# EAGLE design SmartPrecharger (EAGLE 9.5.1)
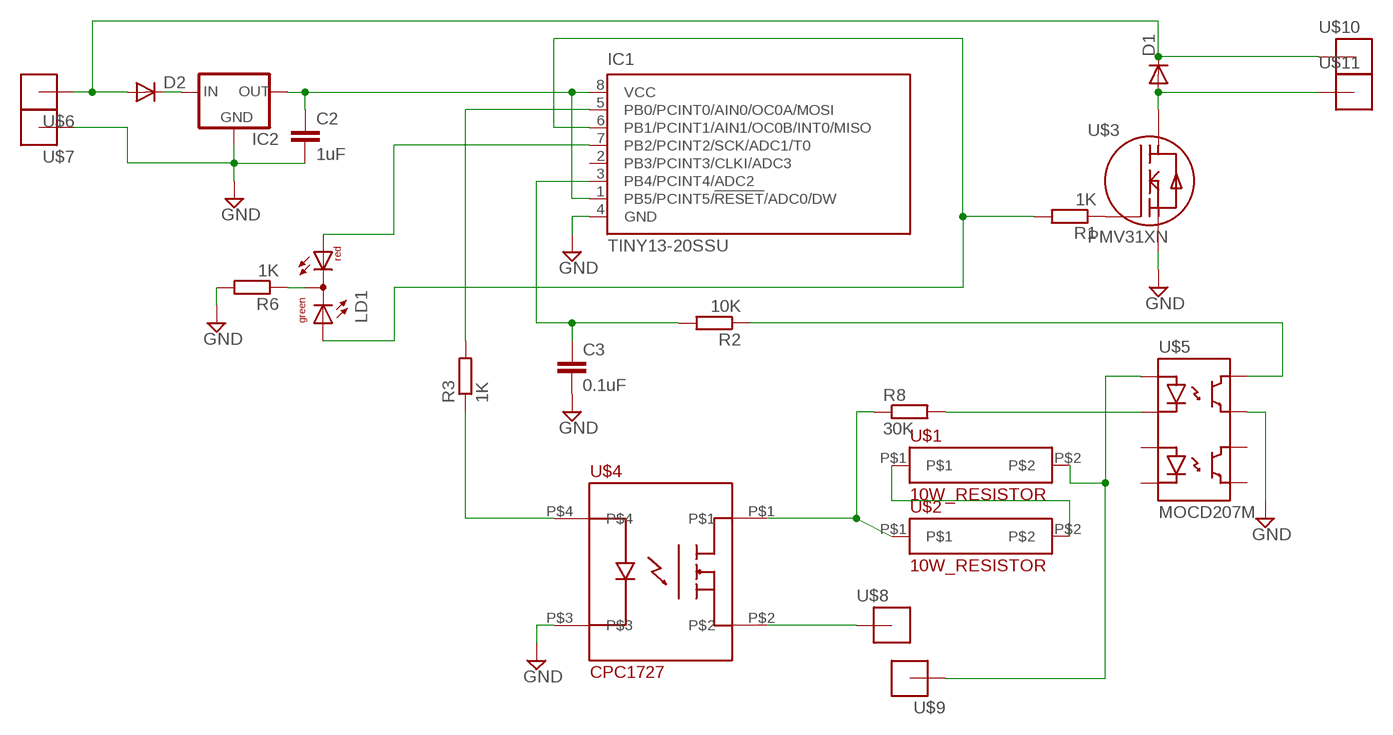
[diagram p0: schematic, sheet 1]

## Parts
C2  1uF  C-EUC1206  [C1206]
C3  0.1uF  C-EUC1206  [C1206]
D1  DIODE-SOD123  [SOD123]
D2  DIODE-SOD123  [SOD123]
IC1  TINY13-20SSU  [8S1]
IC2  78LXXSOT89  [SOT89R]
LD1  DUOLED-RG-C  [DUOLED-C-5MM]
R1  1K  R-EU_R1206  [R1206]
R2  10K  R-EU_R1206  [R1206]
R3  1K  R-EU_R1206  [R1206]
R6  1K  R-EU_R1206  [R1206]
R8  30K  R-EU_R2512  [R2512]
U$1  10W_RESISTOR  [10W_RESISTOR]
U$2  10W_RESISTOR  [10W_RESISTOR]
U$3  PMV31XN  [SOT23]
U$4  CPC1727  [CPC1727]
U$5  MOCD207M  [SOIC8]
U$6  TAB_CONNECTOR  [TAB_CONNECTOR]
U$7  TAB_CONNECTOR  [TAB_CONNECTOR]
U$8  TAB_CONNECTOR  [TAB_CONNECTOR]
U$9  TAB_CONNECTOR  [TAB_CONNECTOR]
U$10  TAB_CONNECTOR  [TAB_CONNECTOR]
U$11  TAB_CONNECTOR  [TAB_CONNECTOR]

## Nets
GND: C2.2 C3.2 IC1.4(GND) IC2.4(GND) R6.2 U$3.P$2(S) U$4.P$3 U$5.P$7(EMITTER1) U$7.P$1
N$1: R2.1 U$5.P$8(COLLECTOR1)
N$2: D2.C IC2.1(IN)
N$3: U$4.P$2 U$8.P$1
N$4: U$1.P$2 U$5.P$1(ANODE1) U$9.P$1
N$5: R8.1 U$2.P$1 U$4.P$1
N$6: R8.2 U$5.P$2(CATHODE1)
N$7: D1.A U$3.P$3(D) U$11.P$1
N$9: C3.1 IC1.3(PB4/PCINT4/ADC2) R2.2
N$10: D1.C D2.A U$6.P$1 U$10.P$1
N$11: R3.1 U$4.P$4
N$12: IC1.5(PB0/PCINT0/AIN0/OC0A/MOSI) R3.2
N$13: R1.1 U$3.P$1(G)
N$15: IC1.6(PB1/PCINT1/AIN1/OC0B/INT0/MISO) LD1.AX(AG) R1.2
N$16: IC1.7(PB2/PCINT2/SCK/ADC1/T0) LD1.AR
N$17: U$1.P$1 U$2.P$2
N$18: C2.1 IC1.1(PB5/PCINT5/!RESET!/ADC0/DW) IC1.8(VCC) IC2.2(OUT)
N$19: LD1.C R6.1
Unconnected: IC1.2(PB3/PCINT3/CLKI/ADC3) U$5.P$3(ANODE2) U$5.P$4(CATHODE2) U$5.P$5(EMITTER2) U$5.P$6(COLLECTOR2)

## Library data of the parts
C2 C3 = resistor:C-EU: CAPACITOR, European symbol
D1 D2 = diode:DIODE-: DIODE
IC1 = atmel:TINY13: 8-bit AVR Microcontroller with 1K Bytes In-System Programmable Flash Source: http://www.atmel.com/dyn/resources/prod_documents/2535S.pdf
IC2 = v-reg:78LXX: VOLTAGE REGULATOR
LD1 = led:DUOLED-RG-C: DUO LED 2 colors (red/green), 5 mm, round, common Cathode www.ligitek.com or other producers.
R1-R3 R6 R8 = resistor:R-EU_: RESISTOR, European symbol
U$1 U$2 = Ians parts:10W_RESISTOR
U$3 = Ians parts:PMV31XN
U$4 = Ians parts:CPC1727
U$5 = Ians parts:MOCD207M
U$6-U$11 = Ians parts:TAB_CONNECTOR

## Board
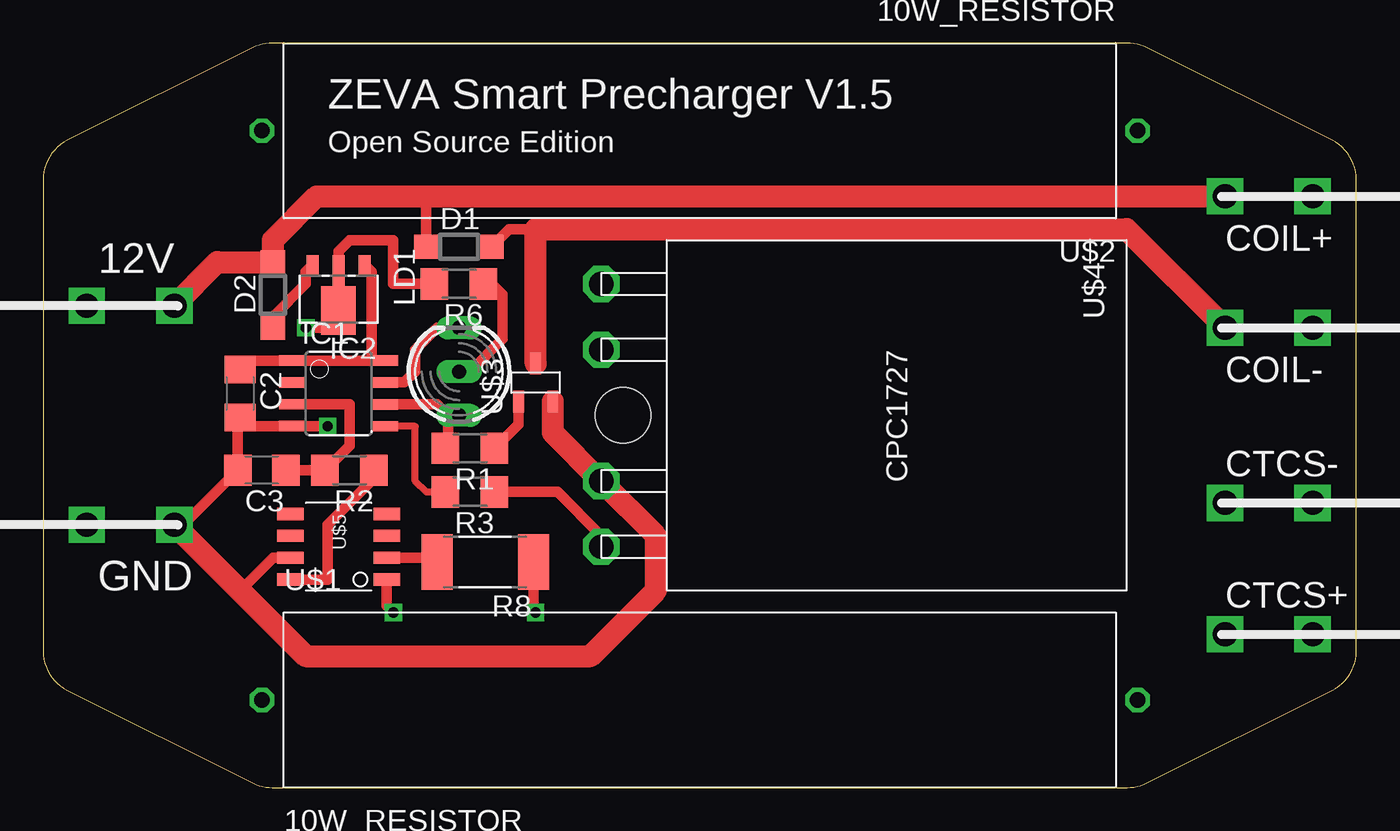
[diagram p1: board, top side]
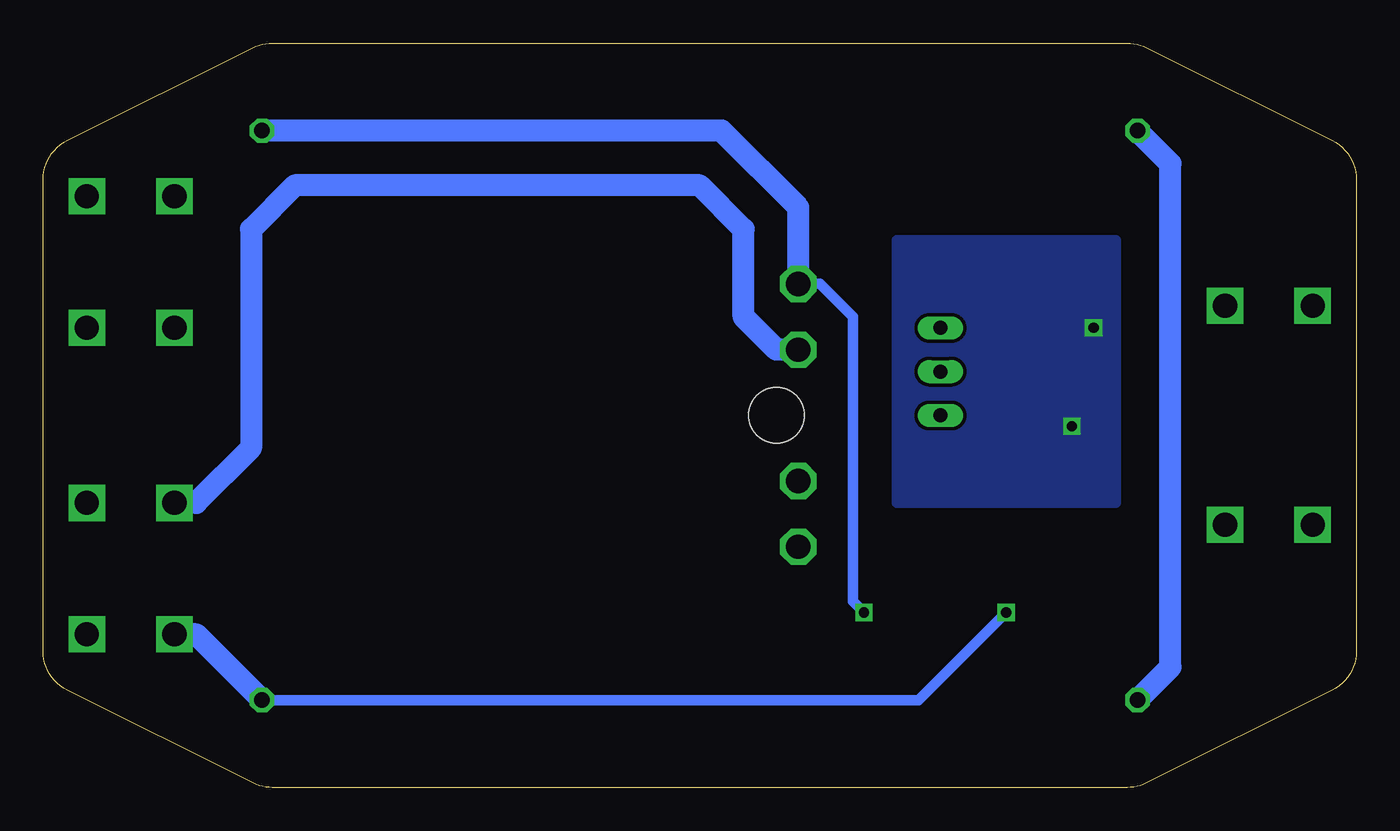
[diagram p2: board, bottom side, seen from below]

Size 76.2 x 43.18 mm. Coordinates in mm from the lower left corner, seen from the top.
Outline: 74.8,5.65 arc63 76.2,7.92 76.2,35.26 arc63 74.8,37.53 64.04,42.91 arc27 62.9,43.18 13.3,43.18 arc27 12.16,42.91 1.4,37.53 arc63 0,35.26 0,7.92 arc63 1.4,5.65 12.16,0.27 arc27 13.3,0 62.9,0 arc27 64.04,0.27 74.8,5.65
Copper layers (1*16): Top 0.035mm / dielectric 1.5mm / Bottom 0.035mm
Design rules "default": minimum track width 10mil, minimum drill 24mil, track to track 8mil, track to pad 8mil, pad to pad 8mil, via to via 8mil, smd to smd 8mil, copper to edge 40mil, drill to drill 8mil, minimum pad ring 10mil, minimum via ring 8mil, stop-mask expansion 4mil, vias tented up to drill 0mil, thermal gap 10mil
Holes 3.2 mm at 33.66,21.59

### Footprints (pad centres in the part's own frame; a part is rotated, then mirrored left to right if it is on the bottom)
C1206 = smd 1.6 x 1.8: 1 -1.4,0; 2 1.4,0
SOD123 = smd 1.4 x 1.4: A 1.9,0; C -1.9,0
8S1 = smd 0.6 x 1.6: 1 -1.905,-2.654; 2 -0.645,-2.654; 3 0.625,-2.654; 4 1.895,-2.654; 5 1.905,2.654; 6 0.635,2.654; 7 -0.635,2.654; 8 -1.905,2.654
SOT89R = smd 0.7 x 1.1: 1 1.5,-1.75; 2 -1.5,-1.75 | smd 0.7 x 1.8: 3 0,-1.4 | smd 2 x 2.8: 4 0,0.9
DUOLED-C-5MM = drill 0.813 long: AR 2.54,0; AX -2.54,0; C 0,0
R1206 = smd 1.6 x 1.803: 1 -1.422,0; 2 1.422,0
R2512 = smd 1.8 x 3.2: 1 -2.8,0; 2 2.8,0
10W_RESISTOR = drill 0.9 octagon: P$1 -25.4,0; P$2 25.4,0
SOT23 = smd 1.27 x 0.635: P$1 -1.1,1; P$2 -1.1,-1; P$3 1.1,0
CPC1727 = drill 1.4 octagon: P$1 -7.62,-16.51; P$2 -3.81,-16.51; P$3 3.81,-16.51; P$4 7.62,-16.51
SOIC8 = smd 1.524 x 0.711: P$1 -2.794,1.905; P$2 -2.794,0.635; P$3 -2.794,-0.635; P$4 -2.794,-1.905; P$5 2.794,-1.905; P$6 2.794,-0.635; P$7 2.794,0.635; P$8 2.794,1.905
TAB_CONNECTOR = drill 1.4 square: P$1 0,2.54; P$2 0,-2.54

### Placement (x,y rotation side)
C2  11.43,22.86 270 top
C3  12.7,18.41 180 top
D1  24.13,31.37 0 top
D2  13.34,28.57 90 top
IC1  17.14,22.86 270 top
IC2  17.14,28.57 180 top
LD1  24.13,24.13 90 top
R1  24.77,19.68 180 top
R2  17.78,18.41 180 top
R3  24.77,17.14 180 top
R6  24.13,29.21 180 top
R8  25.65,13.08 180 top
U$1  38.1,5.08 0 top
U$2  38.1,38.1 180 top
U$3  28.57,23.5 90 top
U$4  48.9,21.59 270 top
U$5  17.14,13.97 180 top
U$6  5.08,27.94 270 top
U$7  5.08,15.24 270 top
U$8  71.12,16.51 90 top
U$9  71.12,8.89 90 top
U$10  71.12,34.29 90 top
U$11  71.12,26.67 90 top

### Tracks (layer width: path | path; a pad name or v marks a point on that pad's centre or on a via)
GND  (via drill 0.6)
  Top 0.61: 11.3,20.96 IC1.4 16.5,20.96 v16.51,20.95 | 11.3,20.96 C3.2 8.12,15.24 U$7.P$1 | C2.2 11.43,21.09 11.3,20.96 | v15.24,26.67 17.14,26.67 IC2.4 17.14,31.11 17.78,31.75 20.32,31.75 20.32,29.21 R6.2 | U$5.P$7 13.34,13.34 11.43,11.43
  Top 1.27: U$7.P$1 11.43,11.43 15.24,7.62 31.75,7.62 35.56,11.43 35.56,14.61 U$4.P$3 29.57,20.59 U$3.P$2
  pour Bottom: 13.97,31.75 26.67,31.75 26.67,16.51 13.97,16.51
N$1
  Top 0.61: R2.1 19.2,17.93 16.51,15.24 16.51,12.06 U$5.P$8
N$2
  Top 0.61: IC2.1 15.24,29.92 15.24,29.21 13.34,27.3 D2.C
N$3
  Bottom 1.27: U$8.P$1 67.31,16.51 64.14,19.68 64.14,32.38 61.59,34.92 38.1,34.92 35.56,32.38 35.56,27.3 33.66,25.4 U$4.P$2
N$4  (via drill 0.6)
  Top 0.61: U$5.P$1 19.94,10.54 v20.32,10.16
  Bottom 0.61: U$1.P$2 25.4,5.08 v20.32,10.16
  Bottom 1.27: U$9.P$1 67.31,8.89 U$1.P$2
N$5  (via drill 0.6)
  Top 0.61: R8.1 28.45,10.28 v28.57,10.16
  Bottom 0.61: U$4.P$1 31.11,29.21 29.21,27.3 29.21,10.79 v28.57,10.16
  Bottom 1.27: U$2.P$1 36.83,38.1 32.38,33.66 U$4.P$1
N$6
  Top 0.61: U$5.P$2 21.96,13.34 R8.2
N$7
  Top 0.61: D1.A 27.05,32.38 28.57,32.38
  Top 1.27: U$3.P$3 28.57,32.38 62.87,32.38 U$11.P$1
N$9
  Top 0.61: C3.1 R2.2 17.78,19.84 17.78,22.23 17.77,22.23 IC1.3
N$10
  Top 0.61: D1.C 22.23,32.01 22.23,34.29
  Top 1.27: U$6.P$1 10.12,30.48 D2.A 13.34,31.75 15.88,34.29 22.23,34.29 U$10.P$1
N$11
  Top 0.61: R3.1 29.84,17.14 32.38,14.61 U$4.P$4
N$12
  Top 0.406: IC1.5 21.59,20.95 21.59,17.78 22.23,17.14 R3.2
N$13
  Top 0.61: U$3.P$1 27.57,21.07 R1.1
N$15
  Top 0.61: IC1.6 22.86,22.23 23.5,21.59 | 23.5,21.59 23.5,19.84 R1.2 | 23.5,21.59 LD1.AX
N$16
  Top 0.61: IC1.7 20.95,23.5 21.59,24.13 21.59,25.4 22.86,26.67 LD1.AR
N$17
  Bottom 1.27: U$2.P$2 10.79,36.2 10.79,6.99 U$1.P$1
N$18
  Top 0.61: C2.1 12.06,24.77 IC1.1 19.05,24.77 | 19.05,24.77 IC1.8 | IC2.2 19.05,29.92 19.05,24.77
N$19
  Top 0.61: R6.1 26.19,29.06 26.67,28.57 26.67,26.04 24.77,24.13 LD1.C

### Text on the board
tPlace: ZEVA Smart Precharger V1.5 | Open Source Edition | COIL+ | 12V | COIL- | CTCS- | GND | CTCS+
